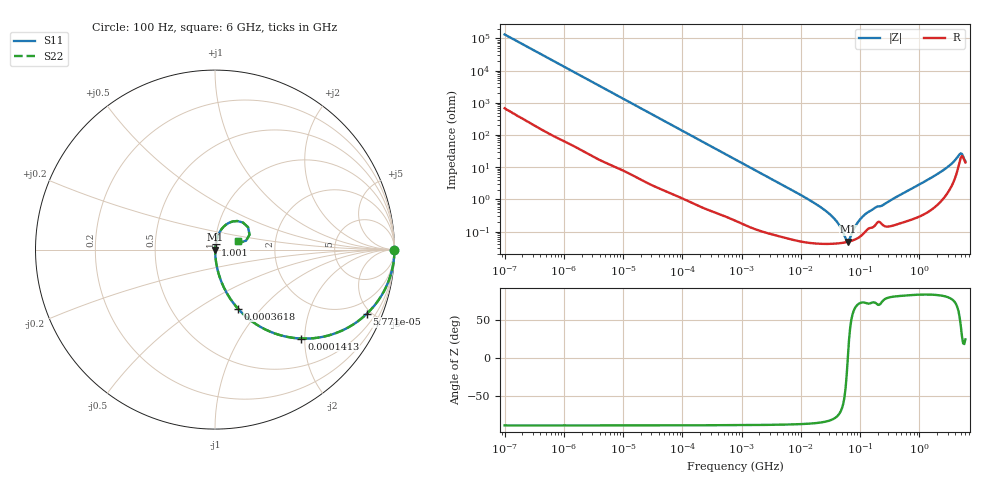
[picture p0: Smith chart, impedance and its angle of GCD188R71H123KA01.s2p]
!Murata Part Number: GCD188R71H123KA01
!These Parameters are Measured in Series Mode Connection
!Data Generated on Jan 08, 2026
!  o--ll--o
!Port1  Port2
!  o------o
!Operation Temp=25[degC], DC Bias Voltage=0[V]
!Freq. Start=100[Hz] Stop=6[GHz] 401[Steps]
# Hz S RI R 50
!Freq.(Hz) S11(Real) S11(Imag) S21(Real) S21(Imag) S12(Real) S12(Imag) S22(Real) S22(Imag)
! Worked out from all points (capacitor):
!   401 points, 100 Hz to 6 GHz, reference 50 ohm
!   read as one part in series: C = 12 nF near 109 Hz
!   lowest |Z| = 48 mohm at 62.33 MHz (marker M1)
!   series resonance near 62.1 MHz, so ESL is about 550 pH
!   S11 on the Smith chart (normalised r, x): 100 Hz: open; 57.71 kHz: 1.03, -4.70; 141.3 kHz: 1.02, -1.93; 361.8 kHz: 1.01, -0.76; 1.001 GHz: 1.01, +0.06; 6 GHz: 1.28, +0.13
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100  1 -0.000753  4.4e-06 0.000753  4.4e-06 0.000753  1 -0.000753
2008  0.9997 -0.015  0.000299 0.015  0.000299 0.015  0.9997 -0.015
12041  0.9916 -0.0885  0.00843 0.0885  0.00843 0.0885  0.9916 -0.0885
40335  0.9171 -0.2726  0.0829 0.2726  0.0829 0.2726  0.9171 -0.2726
57709  0.845 -0.3584  0.155 0.3584  0.155 0.3584  0.845 -0.3584
141303  0.4819 -0.4956  0.5181 0.4956  0.5181 0.4956  0.4819 -0.4956
361830  0.1277 -0.3287  0.8723 0.3287  0.8723 0.3287  0.1277 -0.3287
774597  0.0326 -0.1715  0.9674 0.1715  0.9674 0.1715  0.0326 -0.1715
2481164  0.00404 -0.0555  0.996 0.0555  0.996 0.0555  0.00404 -0.0555
1.555665e7  0.000506 -0.00846  0.9995 0.00846  0.9995 0.00846  0.000506 -0.00846
3.64232e7  0.000426 -0.00253  0.9996 0.00253  0.9996 0.00253  0.000426 -0.00253
4.556224e7  0.000437 -0.00143  0.9996 0.00143  0.9996 0.00143  0.000437 -0.00143
5.699437e7  0.000463 -0.00039  0.9995 0.00039  0.9995 0.00039  0.000463 -0.00039
6.233367e7  0.00048 1.78e-05  0.9995 -1.78e-05  0.9995 -1.78e-05  0.00048 1.78e-05
6.817316e7  0.000501 0.000427  0.9995 -0.000427  0.9995 -0.000427  0.000501 0.000427
8.918374e7  0.000611 0.0017  0.9994 -0.0017  0.9994 -0.0017  0.000611 0.0017
1.166697e8  0.000907 0.00309  0.9991 -0.00309  0.9991 -0.00309  0.000907 0.00309
3.124326e8  0.00152 0.00876  0.9985 -0.00876  0.9985 -0.00876  0.00152 0.00876
1.000774e9  0.00373 0.0287  0.9963 -0.0287  0.9963 -0.0287  0.00373 0.0287
3.205649e9  0.03 0.1043  0.97 -0.1043  0.97 -0.1043  0.03 0.1043
4.796499e9  0.1554 0.151  0.8446 -0.151  0.8446 -0.151  0.1554 0.151
6e9  0.1261 0.0498  0.8739 -0.0498  0.8739 -0.0498  0.1261 0.0498
